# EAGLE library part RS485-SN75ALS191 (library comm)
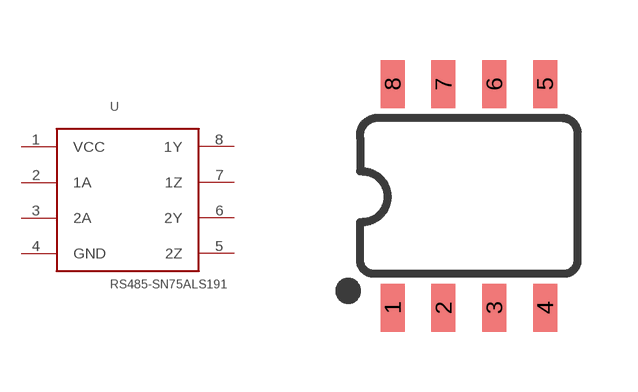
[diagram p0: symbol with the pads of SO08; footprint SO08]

Designator prefix U

## RS485-SN75ALS191SOIC8  [SO08]
1  VCC
2  1A
3  2A
4  GND
5  2Z
6  2Y
7  1Z
8  1Y

## Footprint SO08 (pad centres in mm)
SOIC, 0.15 inch width
smd 0.6 x 1.2: 1 -1.905,-2.8; 2 -0.635,-2.8; 3 0.635,-2.8; 4 1.905,-2.8; 5 1.905,2.8; 6 0.635,2.8; 7 -0.635,2.8; 8 -1.905,2.8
